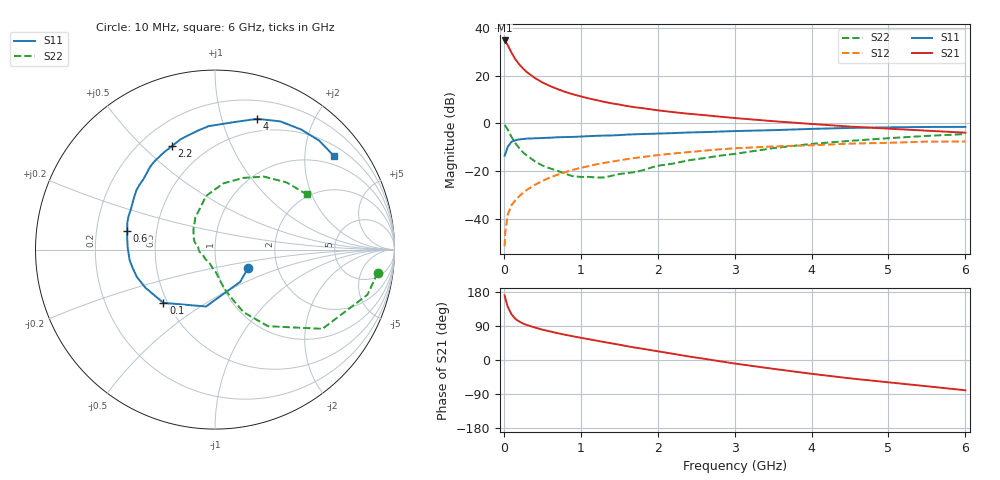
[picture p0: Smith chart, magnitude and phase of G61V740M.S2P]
! SIEMENS Small Signal Semiconductors
! BFG193
! Si NPN RF Bipolar Junction Transistor in SOT223
! VCE = 1.75 V  IC = 40 mA
! Common Emitter S-Parameters:  August  1996
# GHz  S  MA  R  50
!  f  S11  S21  S12  S22
! GHz  MAG  ANG  MAG  ANG  MAG  ANG  MAG  ANG
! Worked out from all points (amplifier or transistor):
!   36 points, 10 MHz to 6 GHz, reference 50 ohm
!   highest |S21| = 34.7 dB at 10 MHz (marker M1)
!   |S21| within 3 dB of that: start of sweep to 66.49 MHz
!   unconditionally stable (mu >= 1): 419.8 MHz to 2.626 GHz
!   at 250 MHz: K = 0.90, MSG = 25.9 dB, |S12| = -29.0 dB
!   at 1.4 GHz: K = 1.06, MAG = 10.7 dB, |S12| = -16.1 dB
!   at 6 GHz: K = 0.93, MSG = 1.8 dB, |S12| = -7.6 dB
!   S11 on the Smith chart (normalised r, x): 10 MHz: 1.42, -0.30; 100 MHz: 0.47, -0.34; 600 MHz: 0.34, +0.09; 2.2 GHz: 0.33, +0.62; 4 GHz: 0.37, +1.31; 6 GHz: 0.74, +2.69
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0.01  0.2109 -28.8  54.11 170.6  0.0027 86.8  0.9155 -8.1
0.02  0.2281 -52.2  51.98 162.4  0.0055 78.3  0.8858 -16.5
0.05  0.3209 -99.0  43.2 140.6  0.0122 68.6  0.7438 -36.4
0.1  0.4132 -134.1  30 120.5  0.0195 63.4  0.5193 -55.3
0.15  0.4419 -151.2  21.82 108.4  0.0247 62.3  0.3833 -65.5
0.2  0.4612 -160.6  17.13 101.6  0.0299 64.5  0.3033 -69.9
0.25  0.4705 -167.6  13.92 96.3  0.0354 64.7  0.2461 -74.3
0.3  0.4793 -173.1  11.76 92.2  0.0406 66.2  0.2125 -77.3
0.4  0.4863 179.0  8.949 86.0  0.0513 66.2  0.162 -82.4
0.5  0.4937 172.3  7.185 80.1  0.0624 65.2  0.1313 -86.5
0.6  0.5007 167.9  6.031 75.4  0.0737 64.6  0.114 -91.7
0.8  0.5167 158.5  4.53 66.5  0.0953 61.6  0.0879 -106.5
1.1  0.5387 146.4  3.329 55.0  0.1275 56.3  0.076 -134.0
1.3  0.5544 139.4  2.825 47.5  0.1485 52.0  0.0736 -156.2
1.6  0.5816 129.2  2.302 36.5  0.1786 45.1  0.0912 -179.9
2.2  0.6246 112.5  1.716 16.4  0.234 31.1  0.1439 146.2
2.8  0.6722 97.4  1.384 -3.0  0.2857 16.6  0.2097 121.6
3.5  0.7197 81.1  1.11 -23.2  0.3281 -0.9  0.3028 99.5
4  0.7655 72.1  0.971 -36.4  0.3485 -10.7  0.372 82.8
4.5  0.8018 63.0  0.856 -48.4  0.3763 -20.8  0.43 68.3
5.5  0.8399 46.3  0.702 -69.3  0.4148 -43.7  0.5469 43.2
6  0.8433 38.4  0.638 -79.9  0.417 -56.7  0.5962 31.1
